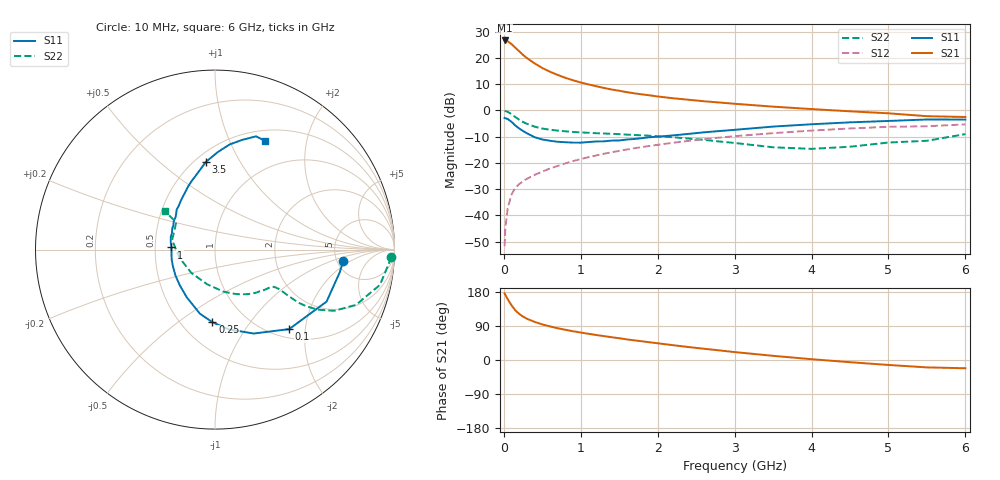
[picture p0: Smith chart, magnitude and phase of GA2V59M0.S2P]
! Infineon Technologies  Discrete & RF Semiconductors
! BF775
! Si NPN RF Bipolar Junction Transistor in SOT23
! VCE = 2.5 V  IC = 9 mA
! Common Emitter S-Parameters:  May  1996
# GHz  S  MA  R  50
!  f  S11  S21  S12  S22
! GHz  MAG  ANG  MAG  ANG  MAG  ANG  MAG  ANG
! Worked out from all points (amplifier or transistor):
!   36 points, 10 MHz to 6 GHz, reference 50 ohm
!   highest |S21| = 26.6 dB at 10 MHz (marker M1)
!   |S21| within 3 dB of that: start of sweep to 158.2 MHz
!   unconditionally stable (mu >= 1): 584.4 MHz to 3.507 GHz
!   at 250 MHz: K = 0.66, MSG = 24.0 dB, |S12| = -27.0 dB
!   at 1.4 GHz: K = 1.12, MAG = 9.8 dB, |S12| = -16.0 dB
!   at 6 GHz: K = 0.97, MSG = 1.4 dB, |S12| = -5.3 dB
!   S11 on the Smith chart (normalised r, x): 10 MHz: 5.63, -1.53; 100 MHz: 1.17, -1.64; 250 MHz: 0.70, -0.68; 1 GHz: 0.61, +0.02; 3.5 GHz: 0.56, +0.73; 6 GHz: 0.63, +1.37
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0.01  0.7165 -5.3  21.43 175.9  0.0026 85.6  0.9829 -2.4
0.02  0.7065 -10.3  21.29 171.7  0.0059 85.0  0.9702 -4.9
0.05  0.6858 -25.0  20.7 160.5  0.0136 77.9  0.9396 -12.1
0.1  0.6057 -47.0  18.28 144.3  0.0251 69.9  0.8437 -21.4
0.15  0.5151 -65.2  15.56 130.9  0.0336 64.2  0.7461 -27.2
0.2  0.4519 -80.0  13.33 121.6  0.0395 61.2  0.6636 -30.3
0.25  0.4047 -92.1  11.36 114.5  0.0449 60.6  0.5999 -31.8
0.3  0.3666 -103.3  9.902 108.8  0.0498 60.4  0.5538 -32.4
0.4  0.3085 -120.8  7.847 100.6  0.0591 60.6  0.4906 -32.3
0.5  0.2794 -134.5  6.399 93.9  0.0683 61.7  0.4507 -31.9
0.6  0.2638 -146.4  5.437 88.6  0.0784 62.2  0.4285 -31.7
0.7  0.2525 -158.0  4.725 83.8  0.0874 62.9  0.4123 -31.7
0.8  0.2476 -167.0  4.166 79.7  0.098 62.9  0.3996 -32.0
1  0.2431 177.1  3.394 72.5  0.1183 62.9  0.3811 -33.1
1.1  0.2496 171.0  3.122 69.2  0.1285 62.3  0.3743 -34.5
1.3  0.2571 158.7  2.671 63.1  0.1492 61.4  0.363 -36.8
1.6  0.279 145.3  2.22 54.4  0.1801 58.9  0.3458 -41.6
2.2  0.3342 124.4  1.701 39.1  0.2419 53.1  0.3078 -53.8
3.5  0.4915 95.9  1.177 11.0  0.3686 37.0  0.1983 -102.6
4.5  0.5919 82.0  0.96 -5.8  0.4524 23.7  0.2033 -167.2
5.5  0.6711 70.1  0.775 -19.5  0.4983 9.1  0.2639 144.9
6  0.6673 65.1  0.748 -21.8  0.5409 5.1  0.3535 142.5
